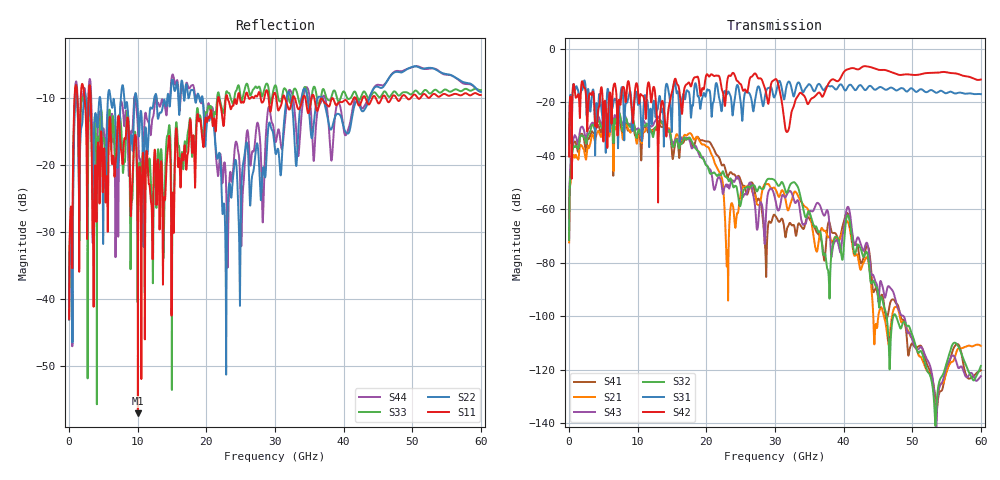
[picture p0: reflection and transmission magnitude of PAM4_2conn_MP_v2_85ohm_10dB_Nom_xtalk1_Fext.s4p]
! Info: Touchstone file created by Circ.  Input file=FAB50GbE_2conn_Midplane_Examax_Topo2_v2_85ohm_10dB_Nom.circ
# Hz S RI R 50
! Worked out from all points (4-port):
!   6000 points, 10 MHz to 60 GHz, reference 50 ohm
!   strongest paths, dB at 10 MHz, 15.01 GHz, 30.01 GHz, 45.01 GHz, 60 GHz:
!     S42: -40.2, -15.9, -11.3, -7.7, -11.4
!     S31: -39.9, -27.1, -17.5, -14.6, -16.9
!     S32: -71.6, -35.8, -49.3, -91.7, -118.7
!     S43: -71.1, -36.3, -55.9, -92.4, -122.5
!     S21: -72.4, -34.9, -52.2, -101.1, -111.2
!     S41: -67.6, -39.3, -62.3, -92.9, -120.3
!   lowest |S11| = -57.1 dB at 10.03 GHz (marker M1), VSWR 1.00, Z = 49.9 - j0.00153 ohm
!   |S11| at or under -10 dB: 3.147 GHz to 21.71 GHz (18.56 GHz wide, 149 % of centre); 23.09 GHz to 24.56 GHz (1.468 GHz wide, 6.16 % of centre); 35.72 GHz to 41.48 GHz (5.757 GHz wide, 14.9 % of centre)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
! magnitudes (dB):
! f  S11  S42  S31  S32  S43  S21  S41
! 10 MHz  -43.0  -40.2  -39.9  -71.6  -71.1  -72.4  -67.6
! 1.02 GHz  -8.1  -18.2  -14.0  -36.2  -33.0  -39.7  -35.4
! 10.03 GHz  -57.1  -15.2  -20.8  -31.0  -29.8  -32.9  -32.0
! 20.26 GHz  -12.9  -9.9  -15.4  -44.4  -44.3  -36.7  -34.6
! 23.05 GHz  -9.8  -11.9  -16.5  -48.4  -51.6  -77.0  -47.8
! 28.81 GHz  -8.9  -17.8  -15.1  -49.1  -57.4  -50.6  -74.9
! 60 GHz  -9.6  -11.4  -16.9  -118.7  -122.5  -111.2  -120.3
